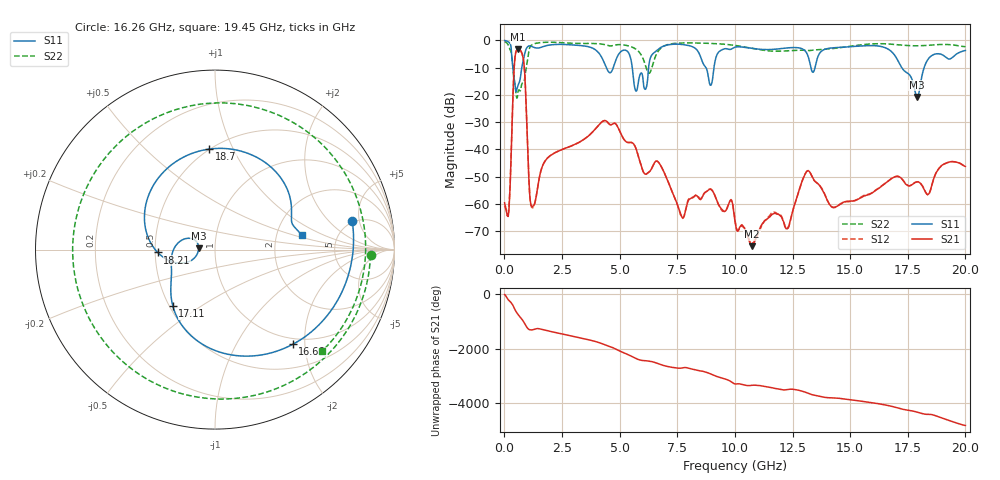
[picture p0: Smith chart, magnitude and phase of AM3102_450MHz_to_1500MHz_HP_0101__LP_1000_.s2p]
!Agilent Technologies,E8364B,MY43040894,A.07.50.67
!Agilent E8364B: A.07.50.67
!Date: Thursday, January 11, 2018 05:41:53
!Correction: S11(Full 2 Port(1,2))
!S21(Full 2 Port(1,2))
!S12(Full 2 Port(1,2))
!S22(Full 2 Port(1,2))
!S2P File: Measurements: S11, S21, S12, S22:
# Hz S  dB  R 50
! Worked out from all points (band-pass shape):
!   1601 points, 10 MHz to 20 GHz, reference 50 ohm
!   highest |S21| = -3.33 dB at 597.2 MHz (marker M1); lowest = -75.6 dB at 10.74 GHz (marker M2)
!   |S21| within 3 dB of the highest: 459.6 MHz to 809.1 MHz (349.5 MHz wide, 55.1 % of centre)
!   lowest |S11| = -20.8 dB at 17.9 GHz (marker M3), VSWR 1.20, Z = 41.7 + j0.677 ohm
!   |S11| at or under -10 dB: 366.5 MHz to 756.2 MHz (389.7 MHz wide, 69.4 % of centre); 5.547 GHz to 6.256 GHz (708.5 MHz wide, 12 % of centre); 17.24 GHz to 18.21 GHz (972.5 MHz wide, 5.49 % of centre)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
!   |S22| runs from -21.2 to -0.5 dB; largest |S21 - S12| = 0.0011
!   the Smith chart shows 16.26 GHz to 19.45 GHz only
!   S11 on the Smith chart (normalised r, x): 16.26 GHz: 4.77, +3.96; 16.66 GHz: 0.89, -1.76; 17.11 GHz: 0.52, -0.39; 18.21 GHz: 0.52, -0.02; 18.7 GHz: 0.50, +0.81; 19.45 GHz: 2.78, +0.59
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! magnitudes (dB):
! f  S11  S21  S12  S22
! 10 MHz  -0.1  -59.6  -60.7  -0.5
! 184.9 MHz  -0.6  -63.4  -62.6  -2.1
! 434.8 MHz  -14.7  -8.8  -8.8  -14.9
! 597.2 MHz  -16.4  -3.3  -3.3  -18.6
! 834.6 MHz  -6.8  -7.6  -7.6  -15.4
! 1.209 GHz  -2.3  -61.0  -61.5  -1.6
! 3.346 GHz  -2.0  -36.9  -36.9  -1.2
! 5.707 GHz  -18.6  -39.7  -39.7  -3.2
! 6.682 GHz  -3.3  -44.7  -44.7  -3.9
! 7.706 GHz  -1.5  -64.9  -65.2  -1.0
! 10.01 GHz  -2.5  -66.4  -65.9  -1.9
! 10.74 GHz  -3.0  -75.6  -74.4  -2.9
! 13.34 GHz  -11.3  -49.9  -49.9  -3.7
! 16.26 GHz  -2.1  -54.2  -54.0  -1.2
! 16.66 GHz  -3.3  -51.6  -51.6  -1.3
! 16.68 GHz  -3.4  -51.5  -51.5  -1.4
! 17.11 GHz  -8.1  -50.0  -50.0  -1.7
! 17.9 GHz  -20.8  -51.9  -51.9  -2.0
! 18.21 GHz  -9.9  -54.8  -54.6  -1.9
! 18.7 GHz  -5.0  -49.1  -49.1  -1.6
! 19.45 GHz  -6.2  -44.5  -44.5  -1.7
! 20 GHz  -3.7  -46.3  -46.3  -2.4
